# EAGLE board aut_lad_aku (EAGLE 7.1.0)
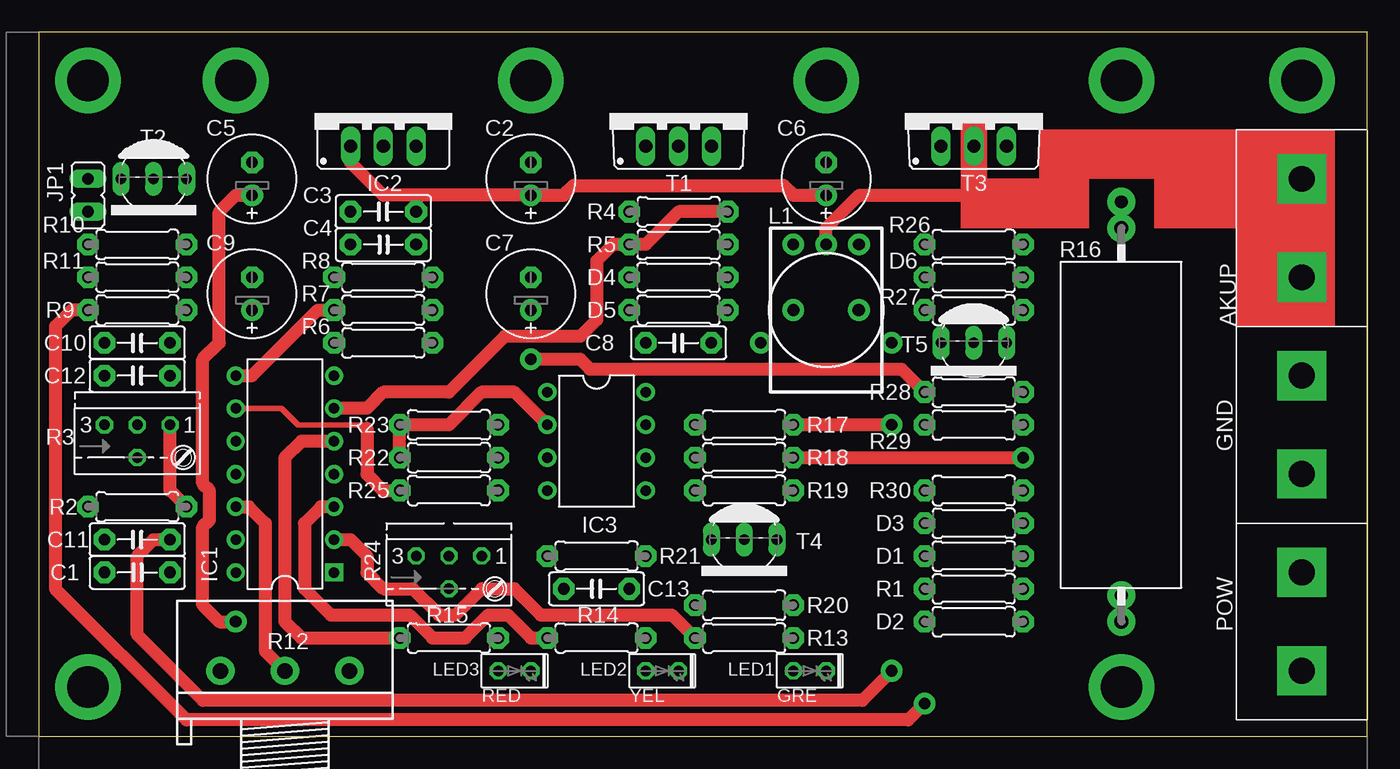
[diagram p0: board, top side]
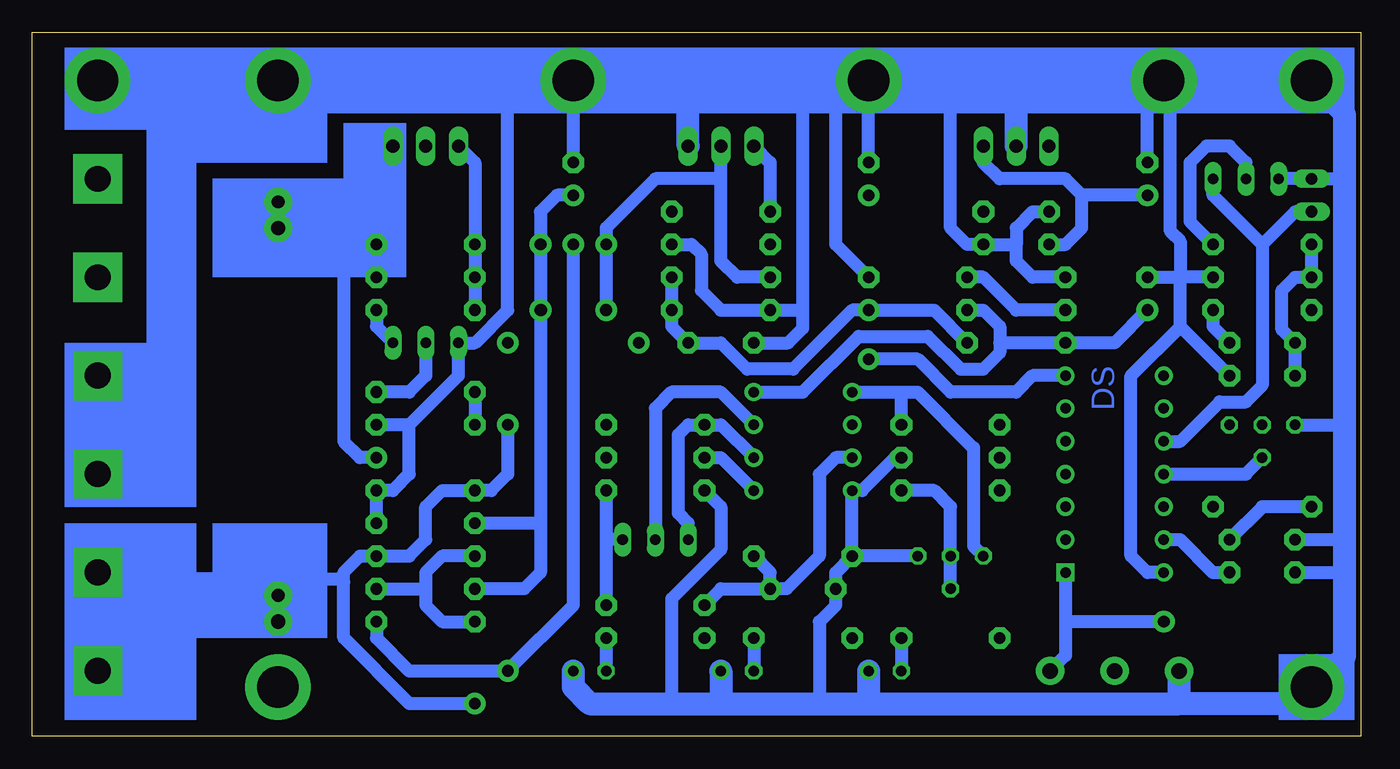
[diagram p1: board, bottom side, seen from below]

Size 102.85 x 54.53 mm. Coordinates in mm from the lower left corner, seen from the top.
Outline: 0,0 102.85,0 102.85,54.53 0,54.53 0,0
Copper layers (1*16): Top 0.035mm / dielectric 1.5mm / Bottom 0.035mm
Design rules "default": minimum track width 10mil, minimum drill 24mil, track to track 8mil, track to pad 8mil, pad to pad 8mil, via to via 8mil, smd to smd 8mil, copper to edge 40mil, drill to drill 8mil, minimum pad ring 10mil, minimum via ring 8mil, stop-mask expansion 4mil, vias tented up to drill 0mil, thermal gap 10mil

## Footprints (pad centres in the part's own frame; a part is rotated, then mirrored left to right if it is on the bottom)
ARK2/750 = drill 2 pad 3.81 square: 1 -3.81,0; 2 3.81,0
C050-025X075 = drill 0.9 pad 1.676 octagon: 1 -2.54,0; 2 2.54,0
E2,5-7 = drill 0.9 pad 1.676: + -1.27,0 | drill 0.9 pad 1.676 octagon: - 1.27,0
0207/7 = drill 0.9 pad 1.676 octagon: 1 -3.81,0; 2 3.81,0
DIL14 = drill 0.813 pad 1.422 square: 1 -7.62,-3.81 | drill 0.813 pad 1.422: 2 -5.08,-3.81; 3 -2.54,-3.81; 4 0,-3.81; 5 2.54,-3.81; 6 5.08,-3.81; 7 7.62,-3.81; 8 7.62,3.81; 9 5.08,3.81; 10 2.54,3.81; 11 0,3.81; 12 -2.54,3.81; 13 -5.08,3.81; 14 -7.62,3.81
78XXS = drill 1.016 long: GND 0,-2.54; IN -2.54,-2.54; OUT 2.54,-2.54
DIL08 = drill 0.813 pad 1.422: 1 -3.81,-3.81; 2 -1.27,-3.81; 3 1.27,-3.81; 4 3.81,-3.81; 5 3.81,3.81; 6 1.27,3.81; 7 -1.27,3.81; 8 -3.81,3.81
JP1 = drill 0.914 long: 1 0,-1.27; 2 0,1.27
6000-XXXX-RC = drill 0.9 pad 1.422: 1 -2.5,0; 2 2.5,0
LED2X5 = drill 0.813 octagon: A -1.27,0; K 1.27,0
S64YW = drill 0.813 octagon: A 2.54,1.27; E -2.54,1.27; S 0,-1.27; S@1 0,1.27
3RP/1610N = drill 1.2 pad 2.184: 1 -5,0; 2 0,0; 3 5,0
VTA52 = drill 1.1 octagon: 1 -15.24,0; 2 15.24,0
TO220BV = drill 1.016 long: D 0,-2.54; G -2.54,-2.54; S 2.54,-2.54
TO92-EBC = drill 0.813 long: B 0,-1.27; C -2.54,-1.27; E 2.54,-1.27

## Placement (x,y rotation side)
AKUP  ARK2  [ARK2/750]  97.79,39.37 90 top
C1  100nF  [C050-025X075]  7.62,15.24 180 top
C2  220/35  [E2,5-7]  38.1,43.18 90 top
C3  100nF  [C050-025X075]  26.67,40.64 180 top
C4  100nF  [C050-025X075]  26.67,38.1 0 top
C5  220/35  [E2,5-7]  16.51,43.18 90 top
C6  220/35  [E2,5-7]  60.96,43.18 90 top
C7  220/35  [E2,5-7]  38.1,34.29 90 top
C8  100nF  [C050-025X075]  49.53,30.48 180 top
C9  220/35  [E2,5-7]  16.51,34.29 90 top
C10  100nF  [C050-025X075]  7.62,30.48 180 top
C11  100nF  [C050-025X075]  7.62,12.7 0 top
C12  100nF  [C050-025X075]  7.62,27.94 180 top
C13  100nF  [C050-025X075]  43.18,11.43 180 top
D1  UF4007  [0207/7]  72.39,13.97 0 top
D2  UF4007  [0207/7]  72.39,8.89 0 top
D3  27V  [0207/7]  72.39,16.51 180 top
D4  UF4007  [0207/7]  49.53,35.56 0 top
D5  33V  [0207/7]  49.53,33.02 0 top
D6  16V  [0207/7]  72.39,35.56 0 top
GND  ARK2  [ARK2/750]  97.79,24.13 90 top
IC1  TINY24  [DIL14]  19.05,20.32 90 top
IC2  7805  [78XXS]  26.67,48.26 0 top
IC3  LM358N  [DIL08]  43.18,22.86 270 top
JP1  [JP1]  3.81,41.91 0 top
L1  100uH  [6000-XXXX-RC]  60.96,33.02 0 top
LED1  GRE  [LED2X5]  59.69,5.08 0 top
LED2  YEL  [LED2X5]  48.26,5.08 0 top
LED3  RED  [LED2X5]  36.83,5.08 0 top
POW  ARK2  [ARK2/750]  97.79,8.89 90 top
R1  1R  [0207/7]  72.39,11.43 0 top
R2  1M  [0207/7]  7.62,17.78 180 top
R3  100k  [S64YW]  7.62,22.86 0 top
R4  47R  [0207/7]  49.53,40.64 180 top
R5  10k  [0207/7]  49.53,38.1 180 top
R6  47R  [0207/7]  26.67,30.48 180 top
R7  100k  [0207/7]  26.67,33.02 0 top
R8  10k  [0207/7]  26.67,35.56 0 top
R9  10k  [0207/7]  7.62,33.02 180 top
R10  10k  [0207/7]  7.62,38.1 180 top
R11  10k  [0207/7]  7.62,35.56 180 top
R12  100k  [3RP/1610N]  19.05,5.08 0 top
R13  1k  [0207/7]  54.61,7.62 0 top
R14  1k  [0207/7]  43.18,7.62 0 top
R15  1k  [0207/7]  31.75,7.62 0 top
R16  2x0.1R  [VTA52]  83.82,24.13 90 top
R17  1k  [0207/7]  54.61,24.13 0 top
R18  1k  [0207/7]  54.61,21.59 0 top
R19  10k  [0207/7]  54.61,19.05 0 top
R20  100k  [0207/7]  54.61,10.16 0 top
R21  1M  [0207/7]  43.18,13.97 0 top
R22  10k  [0207/7]  31.75,21.59 180 top
R23  10k  [0207/7]  31.75,24.13 180 top
R24  100k  [S64YW]  31.75,12.7 0 top
R25  100k  [0207/7]  31.75,19.05 0 top
R26  10k  [0207/7]  72.39,38.1 0 top
R27  1k  [0207/7]  72.39,33.02 180 top
R28  1k  [0207/7]  72.39,26.67 180 top
R29  10k  [0207/7]  72.39,24.13 0 top
R30  10k  [0207/7]  72.39,19.05 0 top
T1  IRF540  [TO220BV]  49.53,48.26 0 top
T2  2N2222  [TO92-EBC]  8.89,41.91 180 top
T3  IRF5305  [TO220BV]  72.39,48.26 0 top
T4  2N2907  [TO92-EBC]  54.61,13.97 180 top
T5  2N2222  [TO92-EBC]  72.39,29.21 180 top

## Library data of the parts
AKUP GND POW = dimmer
C1-C13 D1-D6 L1 R1 R2 R4-R11 R13-R23 R25-R30 = rcl
IC1 = avr-7_2
IC2 = v-reg
IC3 = linear
JP1 = jumper
LED1-LED3 = led
R3 R12 R24 = pot
T1 T3 = transistor-power
T2 T5 = transistor-npn
T4 = transistor-pnp

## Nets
AKUP: AKUP.1 AKUP.2 C1.1 D2.2 R2.2 T3.D
AKUV: IC1.11 R3.S
CV: IC1.9 R25.1
GND: C1.2 C2.- C3.2 C4.2 C5.- C6.- C7.- C8.2 C9.- C11.1 C12.1 C13.2 D3.1 D5.1 GND.1 GND.2 IC1.14 IC2.GND IC3.4 JP1.2 LED1.K LED2.K LED3.K R3.E R5.1 R8.1 R11.1 R12.1 R19.1 R21.1 R22.1 R24.A R29.2 R30.2 T1.S T2.E T5.E
LEDG: IC1.2 R13.1
LEDO: IC1.3 R14.1
LEDR: IC1.5 R15.1
MDR: IC1.7 R28.2 R29.1
N$1: D6.1 R26.1 R27.2 T3.G
N$3: R4.2 T1.G
N$4: D1.1 D2.1 R1.2
N$5: R27.1 T5.C
N$6: C11.2 IC1.13
N$7: IC3.5 R18.1
N$8: C10.2 C12.2 R10.2 R11.2
N$9: IC3.6 R17.1 T4.E
N$10: IC3.7 T4.B
N$11: R19.2 R20.2 T4.C
N$12: R24.S R25.2
N$13: IC3.1 R23.1 R24.E
N$14: C13.1 IC3.3 R20.1 R21.2
N$15: IC3.2 R22.2 R23.2
N$16: D4.1 L1.1 T1.D
N$17: R2.1 R3.A
N$18: R10.1 T2.B
N$19: R28.1 T5.B
N$20: D6.2 R16.2 R18.2 R26.2 T3.S
N$21: C10.1 R9.1
N$22: LED1.A R13.2
N$23: LED2.A R14.2
N$24: LED3.A R15.2
PCV: IC1.8 R7.1 R8.2
PDR: IC1.6 R4.1 R5.2
PMV: C7.+ C8.1 D4.2 D5.2 R6.1
PVCC: C9.+ IC3.8 R6.2 R7.2
REG: IC1.12 R12.2
VCC: C2.+ C3.1 C6.+ D3.2 IC2.IN L1.2 R1.1
VDD: C4.1 C5.+ IC1.1 IC2.OUT R12.3
VIN: D1.2 POW.1 POW.2 R9.2 R16.1 R17.2 R30.1
VIP: IC1.10 JP1.1 T2.C

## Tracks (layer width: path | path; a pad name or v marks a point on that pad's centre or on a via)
AKUP  (via drill 0.9 pad 1.68)
  Top 1.016: T3.D 72.39,41.91 | 72.39,41.91 78.74,41.91 78.74,44.45 97.79,44.45 AKUP.2 AKUP.1 | v60.96,38.1 60.96,39.37 63.5,41.91 72.39,41.91 | v66.04,5.08 63.75,2.79 12.7,2.79 7.62,7.87 7.62,13.97 8.89,15.24 C1.1
  Bottom 1.016: D2.2 76.2,7.62 73.66,5.08 v66.04,5.08 60.96,10.16 v60.96,38.1 | R2.2 7.62,17.78 C1.1
AKUV
  Bottom 1.016: IC1.11 8.89,20.32 R3.S
CV
  Top 0.406: IC1.9 18.8,25.4 20.07,24.13 25.4,24.13 25.4,23.88
  Top 1.016: 25.4,23.88 25.4,20.32 26.67,19.05 R25.1
GND  (via drill 3.2 pad 5.08)
  Bottom 1.016: 43.18,32.77 43.18,50.8 | C2.- v38.1,50.8 | C8.2 44.32,30.48 43.18,31.62 43.18,32.77 | C3.2 25.4,40.64 26.67,39.37 26.67,38.1 | 26.67,38.1 C4.2 30.48,38.1 31.75,39.37 31.75,50.55 31.5,50.8 | C5.- 16.51,50.8 v15.24,50.8 | C6.- v60.96,50.8 | R8.1 25.4,35.56 26.67,36.83 26.67,38.1 | C7.- 40.64,38.1 40.64,50.29 40.13,50.8 | 65.79,50.8 66.04,50.55 66.04,33.02 68.58,30.48 T5.E 69.85,27.94 73.66,24.13 | 43.18,32.77 43.43,33.02 D5.1 49.53,33.02 51.05,34.54 51.05,37.34 51.82,38.1 R5.1 | 73.66,24.13 R29.2 | C9.- 14.22,35.56 13.97,35.31 | 14.73,50.8 14.73,39.12 13.97,38.35 13.97,35.56 | 1.27,43.18 JP1.2 T2.E | R11.1 13.97,35.56 | C1.2 1.27,15.24 | R3.E 1.52,24.13 1.27,24.38 | C11.1 1.52,12.7 1.27,12.95 | IC1.14 16.51,12.7 17.78,13.97 17.78,27.94 13.97,31.75 | 13.97,31.75 13.97,35.31 | 13.97,35.31 13.97,35.56 | 73.66,24.13 73.66,20.32 74.93,19.05 R30.2 D3.1 | R24.A R21.1 | R21.1 40.64,12.7 C13.2 40.64,10.16 41.91,8.89 41.91,2.54 | R21.1 IC3.4 38.61,19.05 36.07,21.59 R22.1 | R19.1 49.53,17.78 49.53,14.48 53.34,10.67 53.34,2.54 | C12.1 13.97,31.75
  Bottom 1.778: 26.67,50.8 31.5,50.8 v38.1,50.8 40.13,50.8 43.18,50.8 52.07,50.8 | 52.07,50.8 v60.96,50.8 65.79,50.8 v83.82,50.8 90.17,50.8 91.44,49.53 91.44,27.94 | IC2.GND 26.67,50.8 | 26.67,50.8 v15.24,50.8 14.73,50.8 v3.81,50.8 1.27,48.26 1.27,43.18 1.27,24.38 1.27,15.24 1.27,12.95 1.27,6.1 5.08,2.54 14.05,2.54 | T1.S 52.07,50.8 | GND.1 91.44,20.32 91.44,27.94 | 91.44,27.94 GND.2 | 14.05,2.54 R12.1 | 49.53,2.54 53.34,2.54 59.69,2.54 60.96,3.81 LED1.K | 49.53,2.54 41.91,2.54 38.1,2.54 | 38.1,2.54 14.05,2.54 | LED2.K 49.53,2.54 | LED3.K 38.1,2.54
LEDG
  Top 1.016: IC1.2 24.13,15.24 25.4,13.97 25.4,12.7 26.67,11.43 28.96,11.43 30.99,9.4 32.26,9.4 34.29,11.43 36.83,11.43 38.86,9.4 49.02,9.4 R13.1
LEDO
  Top 1.016: IC1.3 21.84,17.78 20.57,16.51 20.57,11.43 22.61,9.4 28.7,9.4 30.48,7.62 33.02,7.62 34.8,9.4 36.32,9.4 38.1,7.62 R14.1
LEDR
  Top 1.016: IC1.5 20.32,22.86 19.05,21.59 19.05,8.89 20.32,7.62 R15.1
MDR  (via drill 0.9 pad 1.68)
  Top 1.016: v38.1,29.21 41.91,29.21 42.67,28.45 66.8,28.45 R28.2
  Bottom 1.016: R28.2 R29.1 | IC1.7 25.4,27.94 26.67,26.67 31.75,26.67 34.29,29.21 v38.1,29.21
N$1
  Bottom 1.016: T3.G 68.58,44.45 R26.1 D6.1 R27.2
N$3
  Bottom 1.016: T1.G 45.72,44.45 R4.2
N$4
  Bottom 1.016: 72.39,11.43 72.39,12.7 71.12,13.97 D1.1 | 72.39,11.43 72.39,10.16 71.12,8.89 D2.1 | R1.2 72.39,11.43
N$5
  Bottom 1.016: R27.1 76.2,31.75 T5.C
N$6
  Bottom 1.016: IC1.13 13.97,15.24 11.43,12.7 C11.2
N$7
  Bottom 1.016: R18.1 49.53,21.59 IC3.5
N$8
  Bottom 1.016: R10.2 R11.2 5.08,35.56 6.1,34.54 6.1,31.5 C10.2 C12.2
N$9
  Bottom 1.016: IC3.6 49.53,24.13 R17.1 52.07,24.13 52.83,23.37 52.83,17.27 52.07,16.51 T4.E
N$10
  Bottom 1.016: IC3.7 49.53,26.67 53.34,26.67 54.61,25.4 T4.B
N$11
  Bottom 1.016: R19.2 58.42,15.24 | 58.42,15.24 R20.2 | T4.C 58.42,15.24
N$12
  Bottom 1.016: R24.S 31.75,17.78 33.02,19.05 R25.2
N$13
  Bottom 1.016: R24.E 29.97,14.73 29.97,22.35 34.29,26.67 35.56,26.67 | IC3.1 35.56,26.67 | R23.1 35.56,26.67
N$14
  Bottom 1.016: R20.1 49.53,11.43 C13.1 | C13.1 45.72,12.7 R21.2 | IC3.3 40.64,21.59 41.91,20.32 41.91,13.97 44.45,11.43 C13.1
N$15
  Top 1.016: IC3.2 36.83,26.67 34.29,26.67 31.75,24.13 R23.2 R22.2
N$16  (via drill 0.9 pad 1.68)
  Bottom 1.016: 49.53,43.18 54.61,43.18 58.42,39.37 v58.42,38.1 v58.42,33.02 L1.1 | D4.1 48.26,35.56 49.53,36.83 49.53,43.18 | 49.53,43.18 T1.D
N$17
  Top 1.016: R2.1 10.16,19.05 R3.A
N$18
  Bottom 1.016: T2.B 8.89,44.45 10.16,45.72 11.94,45.72 13.21,44.45 13.21,39.88 R10.1
N$19
  Bottom 1.016: T5.B 72.39,27.94 73.66,26.67 R28.1
N$20  (via drill 0.9 pad 1.68)
  Top 1.016: R18.2 v76.2,21.59
  Bottom 1.016: 76.2,39.37 R26.2 D6.2 | 76.2,39.37 76.2,44.45 T3.S | v76.2,21.59 77.47,21.59 78.74,22.86 78.74,39.12 78.49,39.37 | R16.2 78.49,39.37 | 78.49,39.37 76.2,39.37
N$21
  Bottom 1.016: R9.1 11.43,31.75 C10.1
N$22
  Bottom 1.016: R13.2 LED1.A
N$23
  Bottom 1.016: R14.2 LED2.A
N$24
  Bottom 1.016: R15.2 LED3.A
N$25  (via drill 3.2 pad 5.08)
  other vias: 97.79,50.8
N$26  (via drill 3.2 pad 5.08)
  other vias: 3.81,3.81
N$27  (via drill 3.2 pad 5.08)
  other vias: 83.82,3.81
N$28  (via drill 1 pad 2.18)
  other vias: 83.82,41.4
N$29  (via drill 1 pad 2.18)
  other vias: 83.82,39.37
N$30  (via drill 1 pad 2.18)
  other vias: 83.82,8.89
N$31  (via drill 1 pad 2.18)
  other vias: 83.82,10.92
N$32  (via drill 0.9 pad 1.68)
  other vias: 66.04,30.48
N$33  (via drill 0.9 pad 1.68)
  other vias: 55.88,30.48
PCV
  Top 1.016: IC1.8 16.51,27.94 21.59,33.02 R7.1
  Bottom 1.016: R7.1 26.67,33.02 29.21,35.56 R8.2
PDR
  Top 1.016: R4.1 49.53,40.64 46.99,38.1 R5.2 44.45,38.1 43.18,36.83 43.18,32.26 41.91,30.99 36.07,30.99 31.75,26.67 26.67,26.67 25.4,25.4 IC1.6
PMV
  Bottom 1.016: R6.1 33.02,33.02 C7.+ 39.37,33.02 43.94,28.45 47.5,28.45 49.53,30.48 C8.1 53.34,31.75 D5.2 D4.2
PVCC
  Bottom 1.016: C9.+ 19.05,30.48 R6.2 27.94,30.48 | IC3.8 43.18,26.67 38.86,30.99 33.53,30.99 30.99,28.45 29.21,28.45 27.94,29.72 27.94,30.48 | R7.2 29.21,33.02 27.94,31.75 27.94,30.48
REG
  Top 1.016: IC1.12 16.26,17.78 17.53,16.51 17.53,6.6 R12.2
VCC  (via drill 0.9 pad 1.68)
  Top 1.016: 29.21,41.91 C3.1 | 29.21,41.91 C2.+ 40.64,41.91 41.4,42.67 57.66,42.67 58.42,41.91 C6.+ | 29.21,41.91 26.67,41.91 24.13,44.45 IC2.IN
  Bottom 1.016: 63.5,16.51 63.5,12.7 64.77,11.43 R1.1 | 63.5,16.51 D3.2 | 63.5,16.51 v63.5,33.02 63.46,33.06 L1.2 63.5,33.06 v63.5,38.1 63.5,40.64 62.23,41.91 C6.+
VDD  (via drill 0.9 pad 1.68)
  Top 1.016: C5.+ 15.24,41.91 13.97,40.64 13.97,30.48 12.7,29.21 12.7,19.56 13.21,19.05 13.21,16.76 12.7,16.26 12.7,10.16 13.97,8.89 v15.24,8.89
  Bottom 1.016: C4.1 22.86,38.1 21.59,39.37 21.59,41.91 | C5.+ 21.59,41.91 | v15.24,8.89 22.86,8.89 | 22.86,8.89 22.86,6.27 R12.3 | IC1.1 22.86,8.89 | 21.59,41.91 22.86,43.18 27.94,43.18 29.21,44.45 IC2.OUT
VIN  (via drill 0.9 pad 1.68)
  Top 1.016: v68.58,2.54 67.31,1.27 11.43,1.27 1.27,11.43 1.27,31.75 2.54,33.02 R9.2 | v66.04,24.13 R17.2
  Bottom 1.016: v68.58,2.54 73.66,2.54 78.74,7.62 78.74,11.94 | 78.74,11.94 78.74,12.7 77.47,13.97 D1.2 73.66,13.97 72.39,15.24 72.39,17.78 71.12,19.05 R30.1 67.31,19.05 66.04,20.32 v66.04,24.13 | 78.74,11.94 78.99,12.19 85.09,12.19 R16.1 97.79,8.89 | POW.2 97.79,8.89 | 97.79,8.89 POW.1
VIP
  Bottom 1.016: 7.62,38.1 7.62,27.18 8.89,25.91 10.92,25.91 13.97,22.86 IC1.10 | 7.62,38.1 11.43,41.91 T2.C | JP1.1 5.08,40.64 7.62,38.1
(copper drawn outside any net)
  shapes: Bottom area x15, Top area x6

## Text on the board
Bottom: DS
